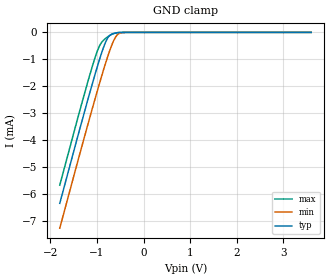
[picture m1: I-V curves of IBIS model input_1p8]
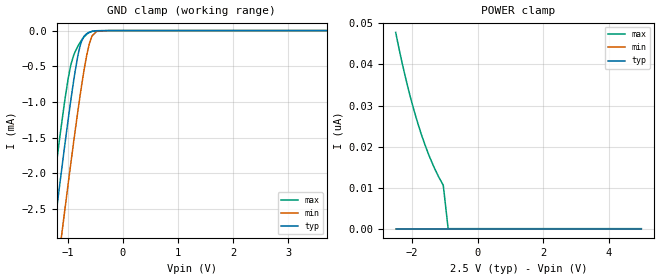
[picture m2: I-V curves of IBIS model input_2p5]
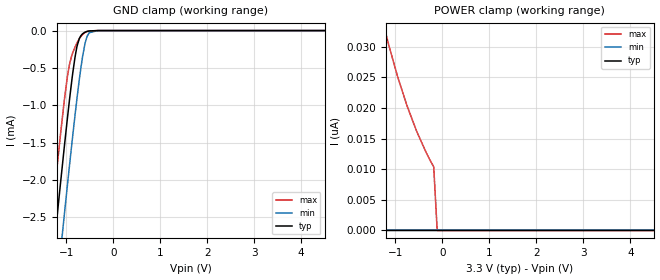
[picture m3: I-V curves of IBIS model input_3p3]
|Texas Instruments Incorporated
| Single Power Supply Inverter Gate CMOS Logic Level Shifter
| Marketing part#   Digital Voltage Range   Package-type   #pins
| SN74LV1T04DBVR   1.6V-5.5V   SOT-23   5
| SN74LV1T04DCKR   1.6V-5.5V   SC70   5
[IBIS Ver]   4.1
[File name]   sn74lv1t04.ibs
[File Rev]   2.0
[Date]   01/23/2014
[Source]
| Texas Instruments Incorporated.
| Analog-eLab Design Center, HPA
| 12500 TI Blvd
| Dallas, TX -75243
[Notes]   Revision History:
| Rev 1.0: 10/25/2007.
| - Initial version of model.
| Rev 1.1: 11/09/2007
| - Power Clamp data dleted as there is no power-clamp diode.
| Rev 2.0: 01/23/2014
| - All new model, wide voltage range based on SN74LV1T00
| - Model generated from simulations in TISPICE
| - Model matched to SPICE simulation
| - C_comp although listed in numerical order of value are
|   obtained from varying PVT conditions. For PVT conditions for
|   each specific value refer the buffer description under
|   respective [Model]. IBIS model user is responsible for using
|   appropriate C_comp to simulate for Signal Integrity.
[Disclaimer]
| This model is designed as an aid for customers of Texas Instruments.
| TI and its licensors and suppliers make no warranties, either expressed
| or implied, with respect to this  model, including the warranties of
| merchantability or fitness for a particular purpose. The model is
| provided solely on an "as is" basis. The entire risk as to its quality
| and performance is with the customer.
[Copyright]
(C) Copyright 2014 Texas Instruments Incorporated.All rights reserved.
|   SN74LV1T04DBVR
[Component]   SN74LV1T04DBVR
[Manufacturer]   TI
[Package]   |5 SOT-23  -  DBV package
|   typ   min   max
R_pkg   0.05933   0.05007   0.06859
L_pkg   1.74585nH   1.48681nH   2.00489nH
C_pkg   0.25506pF   0.25316pF   0.25697pF
[Pin]  signal_name   model_name   R_pin   L_pin   C_pin
1   NC   NC   0.00205   0.92593nH  0.20300pF
2   A   INPUT   0.05007   1.48681nH  0.25697pF
3   GND   GND   0.06861   2.45972nH  0.39612pF
4   Y   OUTPUT   0.06859   2.00489nH  0.25316pF
5   VCC   POWER   0.06799   1.99350nH  0.25166pF
|   SN74LV1T04DCKR
[Component]   SN74LV1T04DCKR
[Manufacturer]   TI
[Package]   |5 SC70   -  DCK package
|   typ   min   max
R_pkg   0.04743   0.04540   0.04946
L_pkg   1.57521nH   1.45465nH   1.69577nH
C_pkg   0.23445pF   0.23255pF   0.23635pF
[Pin]  signal_name   model_name   R_pin   L_pin   C_pin
1   NC   NC   0.00288   0.92487nH  0.18848pF
2   A   INPUT   0.04540   1.45465nH  0.23635pF
3   GND   GND   0.04650   1.67316nH  0.26242pF
4   Y   OUTPUT   0.04946   1.69577nH  0.23255pF
5   VCC   POWER   0.04906   1.68894nH  0.23175pF
|   Model Selectors
[Model Selector] INPUT
input_1p8   1.8V  digital input
input_2p5   2.5V  digital input
input_3p3   3.3V  digital input
input_5p0   5.0V  digital input
[Model Selector] OUTPUT
output_1p8   1.8V  digital output
output_2p5   2.5V  digital output
output_3p3   3.3V  digital output
output_5p0   5.0V  digital output
| Models and submodels in the file (8): input_1p8 (Input), input_2p5 (Input), input_3p3 (Input), input_5p0 (Input), output_1p8 (Output), output_2p5 (Output), output_3p3 (Output), output_5p0 (Output)
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|   input_1p8 Model
[Model]   input_1p8
Model_type   Input
Vinl = 0.58
Vinh = 0.94
|   typ   min   max
|   (nom PVT)   (fast PVT)   (slow PVT)
C_comp   5.699e-13   5.682e-13   5.786e-13
[Model spec]
|subparameter
Vinl   0.58   0.58   0.58
Vinh   0.94   0.94   0.99
| Where nom  PVT is Nominal Process, 1.8V, 40C
|   Fast PVT is Strong Process,  1.98V, -40C
|   Slow PVT is Weak Process,   1.62V, 140C
[Voltage Range]   1.8   1.62   1.98
|Junction Temperature
[Temperature Range]   40   140   -40
[Power Clamp Reference]   1.8   1.62   1.98
[GND Clamp Reference]   0   0   0
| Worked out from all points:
|   GND clamp passes 1 mA (typ) near -0.95 V on its own axis
[GND Clamp]
|   Voltage   I(typ)   I(min)   I(max)
-1.8V     -6.341mA   -7.26mA    -5.666mA
-1.19V    -2.454mA   -3.378mA   -1.786mA
-990.2mV  -1.253mA   -2.152mA   -677.2uA
-899.1mV  -751.6uA   -1.614mA   -367uA
-833.8mV  -437.3uA   -1.242mA   -249.6uA
-775.8mV  -223.4uA   -926.2uA   -169.9uA
-741.6mV  -139.9uA   -749.5uA   -129.6uA
-643.3mV  -37.87uA   -309.6uA   -45.22uA
-604.1mV  -22.25uA   -180.6uA   -25.66uA
-529.9mV  -7.079uA   -43.64uA   -6.907uA
-180mV    0A         -24.71nA   0A
3.6V      0A         0A         0A
[POWER Clamp]
|   Voltage   I(typ)   I(min)   I(max)
-1.8V     0A         0A         0A
0V        0A         0A         0A
3.6V      0A         0A         0A
|   input_2p5 Model
[Model]   input_2p5
Model_type   Input
Vinl = 0.75
Vinh = 1.135
|   typ   min   max
|   (nom PVT)   (fast PVT)   (slow PVT)
C_comp   5.699e-13   5.682e-13   5.751e-13
[Model spec]
|subparameter
Vinl   0.75   0.75   0.75
Vinh   1.135   1.135   1.21
| Where nom  PVT is Nominal Process, 2.5V, 40C
|   Fast PVT is Strong Process,  2.75V, -40C
|   Slow PVT is Weak Process,   2.25V, 140C
[Voltage Range]   2.5   2.25   2.75
|Junction Temperature
[Temperature Range]   40   140   -40
[Power Clamp Reference]   2.5   2.25   2.75
[GND Clamp Reference]   0   0   0
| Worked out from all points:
|   GND clamp passes 1 mA (typ) near -0.95 V on its own axis
[GND Clamp]
|   Voltage   I(typ)   I(min)   I(max)
-2.5V     -10.91mA   -11.81mA   -10.25mA
-1.347V   -3.438mA   -4.365mA   -2.761mA
-1.325V   -3.296mA   -4.223mA   -2.619mA
-1.137V   -2.13mA    -3.051mA   -1.472mA
-1.054V   -1.623mA   -2.535mA   -994.9uA
-945mV    -998uA     -1.883mA   -495.8uA
-817.5mV  -369.4uA   -1.152mA   -225.8uA
-737.5mV  -132.2uA   -728.9uA   -125.2uA
-605.5mV  -22.7uA    -184.6uA   -26.24uA
-472.8mV  -2.598uA   -11.59uA   -2.111uA
-250mV    -24.74nA   -99.19nA   0A
5V        0A         0A         0A
[POWER Clamp]
|   Voltage   I(typ)   I(min)   I(max)
-2.5V     0A         0A         47.81nA
-2.375V   0A         0A         42.98nA
-2.189V   0A         0A         36.44nA
-2V       0A         0A         30.5nA
-1.807V   0A         0A         25.22nA
-1.606V   0A         0A         20.43nA
-1.463V   0A         0A         17.45nA
-1.191V   0A         0A         12.65nA
-1.048V   0A         0A         10.57nA
-899.5mV  0A         0A         0A
5V        0A         0A         0A
|   input_3p3 Model
[Model]   input_3p3
Model_type   Input
Vinl = 0.8
Vinh = 1.35
|   typ   min   max
|   (nom PVT)   (fast PVT)   (slow PVT)
C_comp   5.699e-13   5.665e-13   5.751e-13
[Model spec]
|subparameter
Vinl   0.8   0.8   0.8
Vinh   1.35   1.35   1.47
| Where nom  PVT is Nominal Process, 3.3V, 40C
|   Fast PVT is Strong Process,  3.6V, -40C
|   Slow PVT is Weak Process,   3V, 140C
[Voltage Range]   3.3   3   3.6
|Junction Temperature
[Temperature Range]   40   140   -40
[Power Clamp Reference]   3.3   3   3.6
[GND Clamp Reference]   0   0   0
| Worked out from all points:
|   GND clamp passes 1 mA (typ) near -0.95 V on its own axis
[GND Clamp]
|   Voltage   I(typ)   I(min)   I(max)
-3.3V     -16.17mA   -17.06mA   -15.52mA
-1.623V   -5.197mA   -6.121mA   -4.52mA
-1.251V   -2.832mA   -3.758mA   -2.159mA
-1.126V   -2.057mA   -2.977mA   -1.402mA
-1.04V    -1.54mA    -2.45mA    -920.4uA
-974.4mV  -1.163mA   -2.058mA   -608.3uA
-813mV    -351.6uA   -1.127mA   -219.4uA
-723mV    -108.1uA   -657.3uA   -109.9uA
-594mV    -19.26uA   -153.6uA   -21.87uA
-510mV    -5.045uA   -27.77uA   -4.641uA
-330mV    -154.3nA   -491.7nA   -62.91nA
6.6V      0A         0A         0A
[POWER Clamp]
|   Voltage   I(typ)   I(min)   I(max)
-3.3V     11.07nA    0A         149nA
-3.129V   10.1nA     0A         135nA
-3.044V   0A         0A         128.4nA
-1.345V   0A         0A         36.63nA
-1.168V   0A         0A         31.06nA
-952.8mV  0A         0A         25.11nA
-750mV    0A         0A         20.29nA
-542.4mV  0A         0A         16.09nA
-330mV    0A         0A         12.48nA
-184.8mV  0A         0A         10.39nA
-110.4mV  0A         0A         0A
6.6V      0A         0A         0A
